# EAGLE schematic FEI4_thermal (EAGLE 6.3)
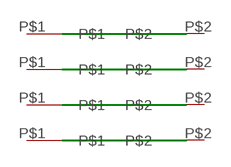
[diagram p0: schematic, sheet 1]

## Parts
U$1  FEI4_THERMAL  [FEI4_THERMAL]
U$2  FEI4_THERMAL  [FEI4_THERMAL]
U$3  FEI4_THERMAL  [FEI4_THERMAL]
U$4  FEI4_THERMAL  [FEI4_THERMAL]
Unconnected: U$1.P$1 U$1.P$2 U$2.P$1 U$2.P$2 U$3.P$1 U$3.P$2 U$4.P$1 U$4.P$2

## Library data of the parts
U$1-U$4 = FE-I4:FEI4_THERMAL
